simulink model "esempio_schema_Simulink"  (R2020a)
settings: Solver=VariableStepAuto  StartTime=0.0  StopTime=30  RelTol=1e-3
undefined symbols (not defined in the file or in its folder): denGs, numGs

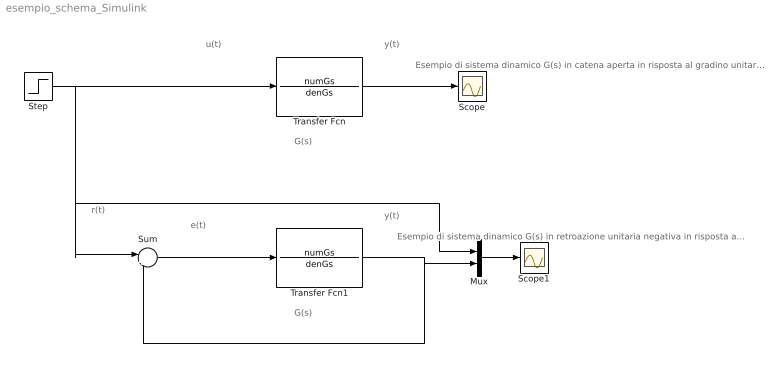
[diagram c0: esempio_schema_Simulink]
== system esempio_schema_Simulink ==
  note: e(t)
  note: Esempio di sistema dinamico G(s) in retroazione unitaria negativa in risposta al gradino
  note: Esempio di sistema dinamico G(s) in catena aperta in risposta al gradino unitario
  note: G(s)
  note: y(t)
  note: u(t)
  note: r(t)
  note: G(s)
  note: y(t)
  Mux : Mux  Inputs=2
  Scope : Scope
  Scope1 : Scope
  Step : Step  Time=0  SampleTime=0
  Sum : Sum  Inputs=|+-
  Transfer Fcn : TransferFcn  Numerator=numGs  Denominator=denGs
  Transfer Fcn1 : TransferFcn  Numerator=numGs  Denominator=denGs
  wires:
  Step/1 -> Mux/1, Sum/1, Transfer Fcn/1
  Transfer Fcn/1 -> Scope/1
  Transfer Fcn1/1 -> Mux/2, Sum/2
  Sum/1 -> Transfer Fcn1/1
  Mux/1 -> Scope1/1
